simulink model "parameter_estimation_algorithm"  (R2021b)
settings: Solver=FixedStepDiscrete  StartTime=0.0  StopTime=10.0  RelTol=1e-3
InitFcn:
  | parameter_estimation_init;
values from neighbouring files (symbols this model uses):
  ADC_resolution = 12    [parameter_estimation_init.m]
  Ts = 1/PWM_frequency    (= 5e-05)    [parameter_estimation_init.m]
undefined symbols (not defined in the file or in its folder): bits, case, DiscIntNeverNeededParam, inverter
libraries: mcbcontrolslib x14, mcbpositiondecoderlib x3, simulink x2
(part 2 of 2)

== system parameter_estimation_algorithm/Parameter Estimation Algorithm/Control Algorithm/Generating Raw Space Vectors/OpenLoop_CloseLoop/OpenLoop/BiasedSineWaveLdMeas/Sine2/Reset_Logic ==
  FeedBack : Inport
  Omega*Ts : Inport  Port=2
  Abs1 : Abs
  Add1 : Sum  Inputs=+-
  Frequency2 : Constant  OutDataTypeStr=single
  Relatioal Operator1 : RelationalOperator  Operator=>
  Unit Delay : UnitDelay  SampleTime=-1  HasFrameUpgradeWarning=on
  Reset : Outport  VectorParamsAs1DForOutWhenUnconnected=off
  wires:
  Omega*Ts/1 -> Add1/2
  Relatioal Operator1/1 -> Unit Delay/1
  FeedBack/1 -> Abs1/1
  Add1/1 -> Relatioal Operator1/2
  Frequency2/1 -> Add1/1
  Abs1/1 -> Relatioal Operator1/1
  Unit Delay/1 -> Reset/1

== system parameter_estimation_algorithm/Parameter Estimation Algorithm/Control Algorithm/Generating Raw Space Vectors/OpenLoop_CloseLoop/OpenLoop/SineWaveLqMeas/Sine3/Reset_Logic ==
  FeedBack : Inport
  Omega*Ts : Inport  Port=2
  Abs1 : Abs
  Add1 : Sum  Inputs=+-
  Frequency2 : Constant  OutDataTypeStr=single
  Relatioal Operator1 : RelationalOperator  Operator=>
  Unit Delay : UnitDelay  SampleTime=-1  HasFrameUpgradeWarning=on
  Reset : Outport  VectorParamsAs1DForOutWhenUnconnected=off
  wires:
  Unit Delay/1 -> Reset/1
  Abs1/1 -> Relatioal Operator1/1
  Frequency2/1 -> Add1/1
  Add1/1 -> Relatioal Operator1/2
  FeedBack/1 -> Abs1/1
  Relatioal Operator1/1 -> Unit Delay/1
  Omega*Ts/1 -> Add1/2

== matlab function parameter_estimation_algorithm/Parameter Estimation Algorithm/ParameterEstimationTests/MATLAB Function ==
function [testNumOut, injFreqOut, refSignalOut, estimatedParameterOut, testEnableOut, estParIdxOut, Kp_iOut, Ki_iOut] = fcn(SignalsPU, Ts, curTime, RsMeasTestTime, I_rated, pole_pairs, Rs, Ld, R_board, V_rated, currentPU_RWV, sigma, IaIbVdc, inverter_V_max, speedFB, speed_rated, Vd_ref_Rs, freqMin, freqMax, freqStep)
%% ************************************************************************
% Function      :   Parameter Estimation Function
% Description   :   Run tests to estimate parameters of PMSM
% Authors       :   H. Gulhane
% Copyright 2020 The MathWorks, Inc.
%% ************************************************************************
coder.allowpcode('plain'); 
%#codegen
[testNumOut, injFreqOut, refSignalOut, estimatedParameterOut, testEnableOut, estParIdxOut, Kp_iOut, Ki_iOut] = mcb.internal.estimateMotorParamAlgoExpo(SignalsPU, Ts, curTime, RsMeasTestTime, I_rated, pole_pairs, Rs, Ld, R_board, V_rated, currentPU_RWV, sigma, IaIbVdc, inverter_V_max, speedFB, speed_rated, Vd_ref_Rs, freqMin, freqMax, freqStep);
